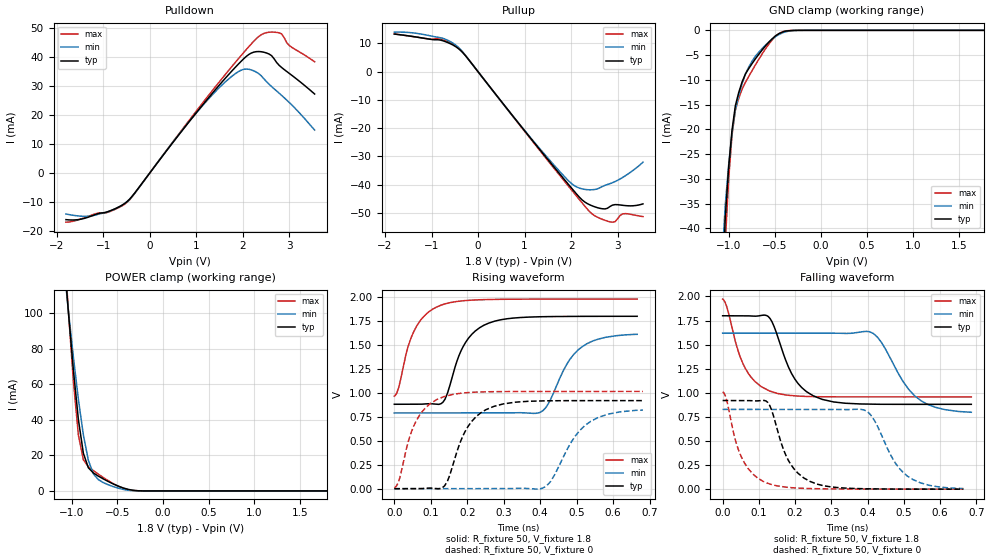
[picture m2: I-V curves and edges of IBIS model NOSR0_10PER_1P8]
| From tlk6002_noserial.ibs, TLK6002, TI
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[Model]   NOSR0_10PER_1P8
Model_type   3-state
Polarity   Non-Inverting
Enable   Active-Low
Cref =  15.0000pF
Rref =  100.0000M
Vref =  0V
Vmeas =  0.9
C_comp   1.885425p   1.715283p   2.176444p
[Temperature Range]   25   125   -40
[Voltage Range]   1.8   1.62   1.98
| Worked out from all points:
|   slope of the pulldown table from 0 to 0.27 V, typ, clamps not added: 47.1 ohm
|   slope of the pullup table from 0 to 0.27 V, typ, clamps not added: 47.4 ohm
|   GND clamp passes 1 mA (typ) near -0.48 V on its own axis
|   POWER clamp passes 1 mA (typ) near -0.39 V on its own axis
|   rising waveform, R_fixture 50, V_fixture 1.8: 20-80 % time 62.2ps typ, 72.4ps min, 57ps max; typ from 0.881 V to 1.8 V
|   rising waveform, R_fixture 50, V_fixture 0: 20-80 % time 64.4ps typ, 79.5ps min, 57.5ps max; typ from 0 V to 0.92 V
|   falling waveform, R_fixture 50, V_fixture 1.8: 20-80 % time 66.5ps typ, 82.8ps min, 58.7ps max; typ from 1.8 V to 0.882 V
|   falling waveform, R_fixture 50, V_fixture 0: 20-80 % time 60.9ps typ, 72.5ps min, 55.1ps max; typ from 0.921 V to 0.002 V
[POWER_clamp]
-1.8V     644.6mA    525mA      777mA
-1.055V   111.8mA    110.1mA    115.1mA
-1.036V   100.1mA    100.9mA    100.7mA
-981.8mV  67.73mA    75.06mA    61.46mA
-927.3mV  40.06mA    51.42mA    31.32mA
-872.7mV  21.16mA    31.46mA    17.47mA
-818.2mV  13.02mA    17.22mA    13.65mA
-763.6mV  10.12mA    9.635mA    11.46mA
-654.5mV  6.765mA    4.687mA    7.551mA
-436.4mV  1.678mA    857.7uA    1.497mA
-272.7mV  101.6uA    39.42uA    61.35uA
1.8V      90.02nA    111.7nA    348.8nA
[Pulldown]
-1.8V     -16mA      -14.06mA   -16.88mA
-1.2V     -14.43mA   -14.55mA   -14.16mA
-490.9mV  -9.876mA   -9.852mA   -10.12mA
1.2V      24.63mA    24.33mA    25.37mA
1.691V    33.76mA    32.26mA    35.17mA
2.018V    39.25mA    35.65mA    41.38mA
2.4V      41.7mA     33.4mA     47.57mA
2.618V    40.38mA    29.76mA    48.46mA
2.727V    38.02mA    28.23mA    48.35mA
2.836V    36.27mA    26.68mA    47.83mA
3V        34.26mA    24.25mA    43.84mA
3.545V    27.17mA    14.78mA    38.26mA
[Pullup]
-1.8V     13.31mA    13.99mA    13.35mA
-763.6mV  10.98mA    11.84mA    11.28mA
-436.4mV  8.351mA    8.806mA    8.623mA
-272.7mV  5.714mA    5.817mA    5.773mA
1.364V    -28.29mA   -27.93mA   -28.62mA
1.909V    -39.21mA   -38.01mA   -39.8mA
2.127V    -43.46mA   -40.83mA   -44.21mA
2.455V    -47.47mA   -41.76mA   -50.35mA
2.782V    -48.32mA   -39.91mA   -52.87mA
2.945V    -47.03mA   -38.87mA   -53.08mA
3.109V    -47.27mA   -37.41mA   -50.31mA
3.545V    -46.77mA   -32.01mA   -51.27mA
[GND_clamp]
-1.8V     -566.4mA   -409.5mA   -760.6mA
-1.073V   -54mA      -46.59mA   -65.57mA
-1.036V   -37.78mA   -35.21mA   -42.82mA
-1V       -27.67mA   -27.21mA   -30.08mA
-963.6mV  -20.15mA   -20.81mA   -21.18mA
-927.3mV  -15.22mA   -16.02mA   -16.11mA
-890.9mV  -12.56mA   -13.16mA   -13.75mA
-818.2mV  -8.811mA   -8.807mA   -10.5mA
-745.5mV  -6.683mA   -6.208mA   -8.112mA
-454.5mV  -667.9uA   -843.5uA   -644.9uA
-236.4mV  -5uA       -16.82uA   -2.48uA
1.764V    74.33nA    1.736uA    140.7nA
[Ramp]
dV/dt_f  0.4628391/52.19683p   0.4238012/68.31142p   0.5111784/45.89154p
dV/dt_r  0.4607535/50.37324p   0.4169442/64.54756p   0.5087354/44.96875p
R_load = 50
[Rising Waveform]
R_fixture = 50
V_fixture = 1.8
V_fixture_min = 1.62
V_fixture_max = 1.98
0s        881.4mV    790.8mV    966mV
58ps      881.2mV    790.8mV    1.675V
126ps     884.4mV    790.8mV    1.913V
145ps     987.1mV    790.8mV    1.936V
194ps     1.519V     790.8mV    1.964V
256ps     1.725V     790.8mV    1.975V
405ps     1.796V     808.4mV    1.98V
471ps     1.798V     1.287V     1.98V
513ps     1.799V     1.477V     1.98V
666ps     1.8V       1.612V     1.98V
[Rising Waveform]
R_fixture = 50
V_fixture = 0
V_fixture_min = 0
V_fixture_max = 0
0s        6.313uV    1.049uV    8.26mV
15ps      9.871uV    1.035uV    112mV
38ps      -19.27uV   1.014uV    488mV
58ps      -196.8uV   994.7nV    692.8mV
136ps     23.82mV    -186.5nV   961.6mV
201ps     643mV      151.7nV    1.003V
270ps     855.7mV    -227.4uV   1.013V
406ps     917mV      4.468mV    1.015V
521ps     919.4mV    654.2mV    1.015V
682ps     919.5mV    820.7mV    1.016V
[Falling Waveform]
R_fixture = 50
V_fixture = 1.8
V_fixture_min = 1.62
V_fixture_max = 1.98
0s        1.8V       1.62V      1.973V
11ps      1.8V       1.62V      1.898V
61ps      1.8V       1.62V      1.265V
128ps     1.784V     1.62V      1.022V
189ps     1.209V     1.62V      972.7mV
249ps     971.3mV    1.62V      961.2mV
415ps     882.4mV    1.618V     958.8mV
530ps     881.4mV    969mV      958.8mV
584ps     881.6mV    853.7mV    958.7mV
686ps     881.7mV    799.2mV    958.7mV
[Falling Waveform]
R_fixture = 50
V_fixture = 0
V_fixture_min = 0
V_fixture_max = 0
0s        920.9mV    828.9mV    1.011V
10ps      920.9mV    828.9mV    940.2mV
51ps      921.1mV    828.9mV    341.1mV
117ps     919.5mV    828.9mV    73.31mV
135ps     823.7mV    828.9mV    49.74mV
180ps     309mV      828.9mV    20.41mV
239ps     85.01mV    828.9mV    7.816mV
391ps     5.82mV     822.1mV    2.657mV
509ps     2.227mV    138.7mV    2.189mV
664ps     1.6mV      8.228mV    1.724mV
